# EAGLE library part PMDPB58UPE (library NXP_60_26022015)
20 V dual P-channel Trench MOSFET Dual small-signal P-channel enhancement mode Field-Effect Transistor (FET) in a leadless medium power DFN2020-6 (SOT1118) Surface-Mounted Device (SMD) plastic package using Trench MOSFET technology. AAL Eindhoven MK
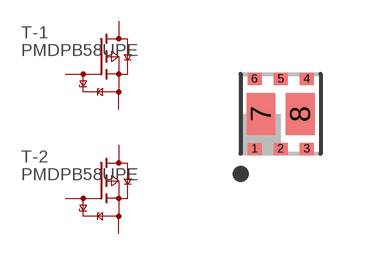
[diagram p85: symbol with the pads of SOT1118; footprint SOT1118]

Designator prefix T; gates -1=P-MOSFER-TR -2=P-MOSFER-TR

## PMDPB58UPE  [SOT1118]
1  -1:S  pas
2  -1:G  pas
3  -2:D  pas
4  -2:S  pas
5  -2:G  pas
6  -1:D  pas
7  -1:D  pas
8  -2:S  pas

## Footprint SOT1118 (pad centres in mm)
SOT1118 HUSON6: plastic, thermal enhanced ultra thin small outline package; no leads;6 terminals; body 2 x 2 x 0.65 mm JEDEC: -- IEC: -- JEITA: --
smd 0.35 x 0.3: 1 -0.65,-0.875; 2 0,-0.875; 3 0.65,-0.875; 4 0.65,0.875; 5 0,0.875; 6 -0.65,0.875
smd 0.72 x 1.05: 7 -0.49,0; 8 0.49,0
